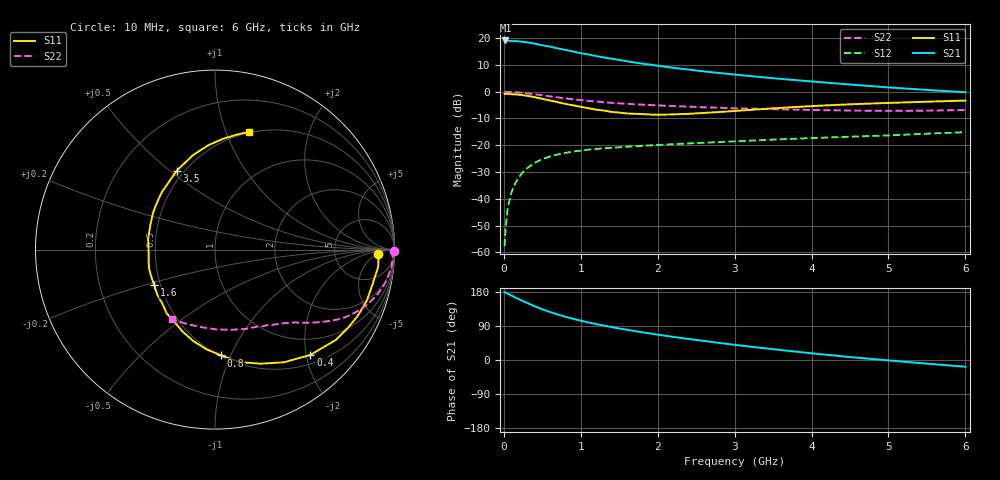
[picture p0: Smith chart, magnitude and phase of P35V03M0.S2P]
! SIEMENS Small Signal Semiconductors
! BFP181
! Si NPN RF Bipolar Junction Transistor in SOT143
! VCE = 5 V  IC = 3 mA
! Common Emitter S-Parameters:  March  1996
# GHz  S  MA  R  50
!  f  S11  S21  S12  S22
! GHz  MAG  ANG  MAG  ANG  MAG  ANG  MAG  ANG
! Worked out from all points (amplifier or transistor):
!   36 points, 10 MHz to 6 GHz, reference 50 ohm
!   highest |S21| = 19.2 dB at 20 MHz (marker M1)
!   |S21| within 3 dB of that: start of sweep to 705.9 MHz
!   unconditionally stable (mu >= 1): 2.171 GHz to end of sweep
!   at 250 MHz: K = 0.16, MSG = 24.3 dB, |S12| = -30.0 dB
!   at 1.4 GHz: K = 0.75, MSG = 16.6 dB, |S12| = -21.0 dB
!   at 6 GHz: K = 1.09, MAG = 5.6 dB, |S12| = -15.1 dB
!   lowest NFmin = 1.40 dB at 450 MHz
!   S11 on the Smith chart (normalised r, x): 10 MHz: 20, -5; 400 MHz: 0.66, -2.08; 800 MHz: 0.51, -0.92; 1.6 GHz: 0.46, -0.22; 3.5 GHz: 0.46, +0.53; 6 GHz: 0.49, +1.21
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0.01  0.9102 -1.5  9.034 178.9  0.0013 84.5  0.9951 -0.4
0.02  0.9117 -2.5  9.073 178.3  0.0024 80.8  0.9904 -1.1
0.05  0.9142 -6.0  8.995 174.8  0.0067 91.6  0.991 -2.8
0.1  0.8987 -12.6  8.844 170.0  0.0133 83.0  0.9884 -5.6
0.15  0.892 -18.8  8.834 164.8  0.0196 78.4  0.977 -8.4
0.25  0.8591 -30.6  8.537 155.1  0.0315 72.3  0.9509 -13.6
0.3  0.8403 -36.8  8.39 151.0  0.0369 69.0  0.9341 -16.0
0.4  0.7917 -47.8  7.913 141.8  0.0468 63.1  0.8985 -20.3
0.5  0.7367 -58.4  7.379 133.8  0.055 58.1  0.8582 -24.0
0.6  0.6844 -68.3  6.969 126.6  0.0616 53.5  0.8195 -27.3
0.8  0.5905 -86.6  6.058 114.1  0.0717 46.6  0.7505 -32.0
1  0.5228 -103.5  5.248 103.8  0.0792 41.6  0.6967 -35.6
1.1  0.4904 -111.8  4.957 99.0  0.0826 39.5  0.6744 -37.1
1.3  0.4454 -127.2  4.366 90.8  0.0876 36.4  0.6366 -39.8
1.6  0.3922 -149.8  3.705 79.7  0.0937 33.4  0.5943 -43.1
1.9  0.3751 -170.7  3.207 70.0  0.0993 30.8  0.5632 -46.7
2.2  0.3773 170.9  2.799 61.0  0.1047 29.2  0.5395 -50.4
2.8  0.417 140.6  2.235 45.0  0.1147 26.5  0.5026 -58.4
3.5  0.489 115.8  1.786 28.5  0.1274 23.7  0.4724 -69.5
4.5  0.5818 93.9  1.361 7.7  0.1441 19.0  0.4449 -89.2
5.5  0.6504 79.6  1.08 -9.7  0.1643 15.3  0.443 -110.4
6  0.6828 73.8  0.976 -17.7  0.1754 12.5  0.4549 -121.4
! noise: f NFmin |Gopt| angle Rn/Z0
0.45  1.4  0.56  17  0.36
0.9  1.5  0.45  35  0.34
1.8  1.85  0.25  82  0.36
